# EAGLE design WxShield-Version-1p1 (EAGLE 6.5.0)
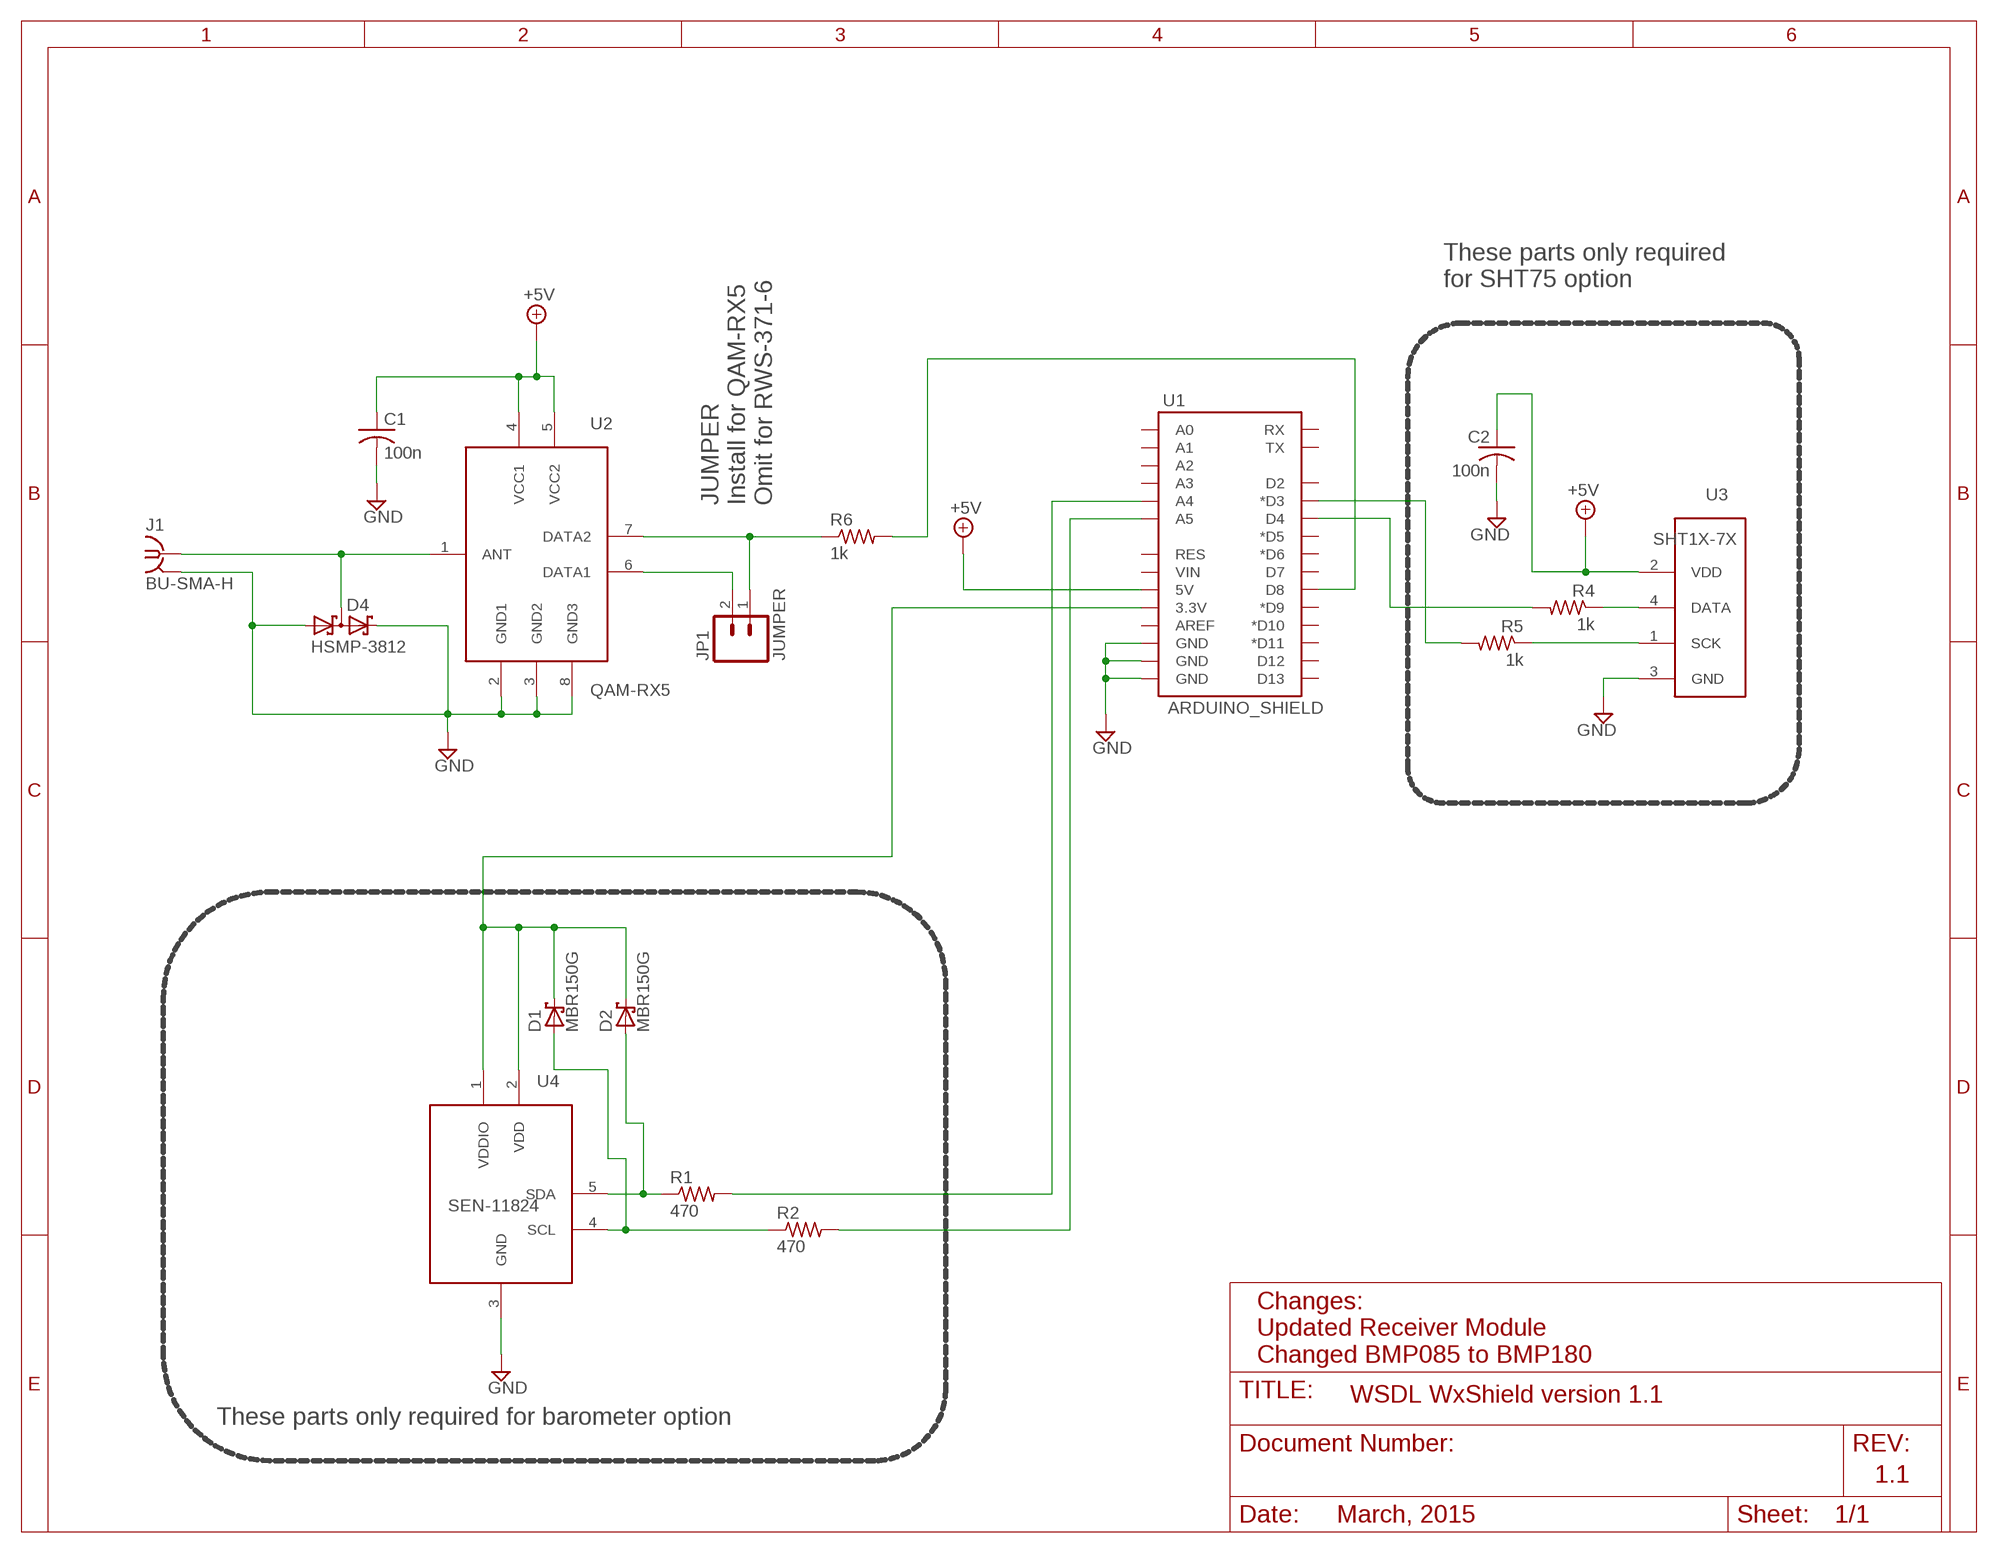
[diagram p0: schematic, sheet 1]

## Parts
C1  100n  C-US050-025X075  [C050-025X075]
C2  100n  C-US050-025X075  [C050-025X075]
D1  MBR150G  1N5817-B  [DO41-7.6]
D2  MBR150G  1N5817-B  [DO41-7.6]
D4  HSMP-3812  BAT30SW  [SOT323]
J1  BU-SMA-H  [BU-SMA-H]
JP1  JUMPER  M021X02_NO_SILK  [1X02_NO_SILK]
R1  470  R-US_0207/10  [0207/10]
R2  470  R-US_0207/10  [0207/10]
R4  1k  R-US_0207/10  [0207/10]
R5  1k  R-US_0207/10  [0207/10]
R6  1k  R-US_0207/10  [0207/10]
U1  ARDUINO_SHIELD  ARDUINO_SHIELDLABEL  [DUEMILANOVE_SHIELD]
U2  QAM-RX5  QAM-RX4  [QAM-RX4]
U3  SHT1X-7X  [SHT7X]
U4  SEN-11824  [SEN-11824]

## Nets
+5V: C1.1 C2.1 U1.5V U2.4(VCC1) U2.5(VCC2) U3.2(VDD)
GND: C1.2 C2.2 D4.1(A1) D4.2(C2) J1.2(GND) U1.GND@0(GND) U1.GND@1(GND) U1.GND@2(GND) U2.2(GND1) U2.3(GND2) U2.8(GND3) U3.3(GND) U4.3(GND)
N$1: JP1.1 R6.1 U2.7(DATA2)
N$2: JP1.2 U2.6(DATA1)
N$3: D2.A R1.1 U4.5(SDA)
N$4: D1.A R2.1 U4.4(SCL)
N$5: R1.2 U1.A4
N$6: R2.2 U1.A5
N$8: R4.1 U3.4(DATA)
N$9: R5.1 U3.1(SCK)
N$10: R5.2 U1.D3(*D3)
N$11: R4.2 U1.D4
N$12: R6.2 U1.D8
N$13: D1.C D2.C U1.3.3V U4.1(VDDIO) U4.2(VDD)
N$19: D4.3(C1A2) J1.1 U2.1(ANT)
Unconnected: U1.A0 U1.A1 U1.A2 U1.A3 U1.AREF U1.D2 U1.D5(*D5) U1.D6(*D6) U1.D7 U1.D9(*D9) U1.D10(*D10) U1.D11(*D11) U1.D12 U1.D13 U1.RES U1.RX U1.TX U1.VIN

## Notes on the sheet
- These parts only required
  for SHT75 option
- JUMPER
  Install for QAM-RX5
  Omit for RWS-371-6
- Changes:
  Updated Receiver Module
  Changed BMP085 to BMP180
- WSDL WxShield version 1.1
- These parts only required for barometer option
- 1.1
- March, 2015

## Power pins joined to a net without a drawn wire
GND: J1.3(GND) J1.4(GND) J1.5(GND)

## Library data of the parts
C1 C2 = resistor:C-US: CAPACITOR, American symbol
D1 D2 = diode:1N581*: 1.0A SCHOTTKY BARRIER RECTIFIER
D4 = max-local:BAT30SW: Dual Schottky diode Available in SOT-323 package
J1 = con-coax:BU-SMA-H: FEMALE SMA CONNECTOR Radiall
JP1 = SparkFun-Connectors:M02: Header 2
R1 R2 R4-R6 = resistor:R-US_: RESISTOR, American symbol
U1 = SparkFun-Boards:ARDUINO_SHIELD: Arduino shield footprint
U2 = max-local:QAM-RX4: RF Solutions OOK Receiver Module
U3 = max-local:SHT1X
U4 = max-local:SEN-11824: SparkFun BMP180 Breakout Board

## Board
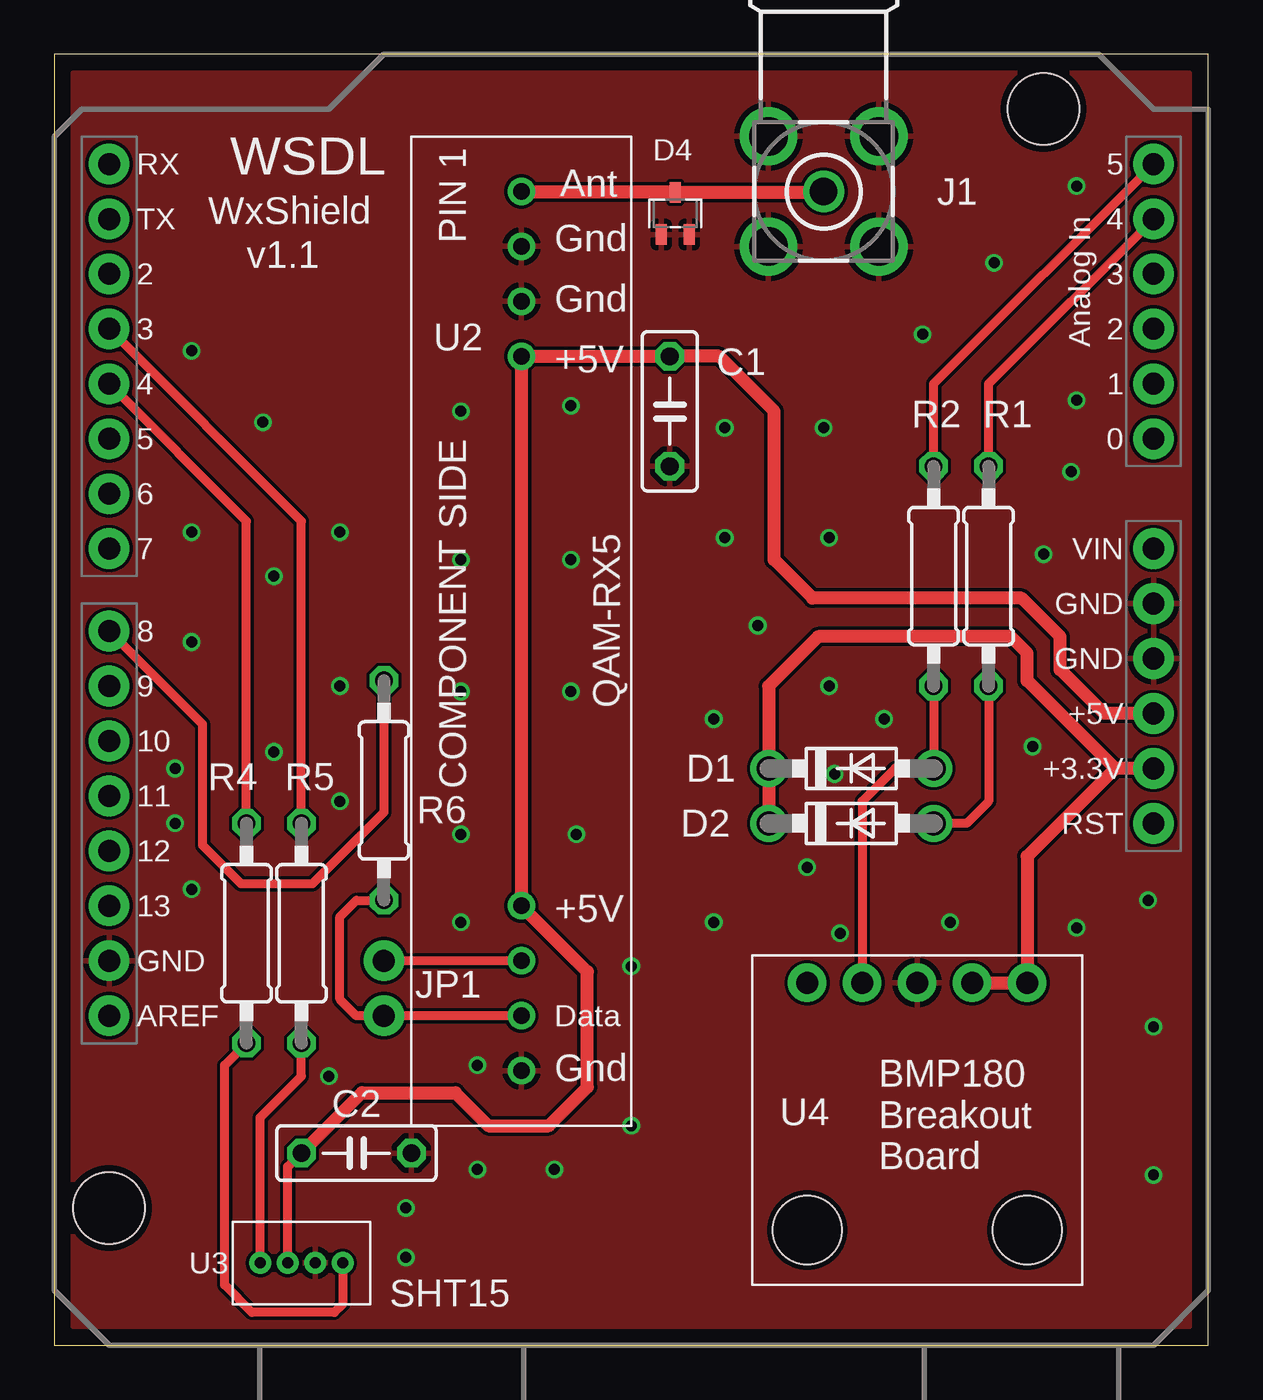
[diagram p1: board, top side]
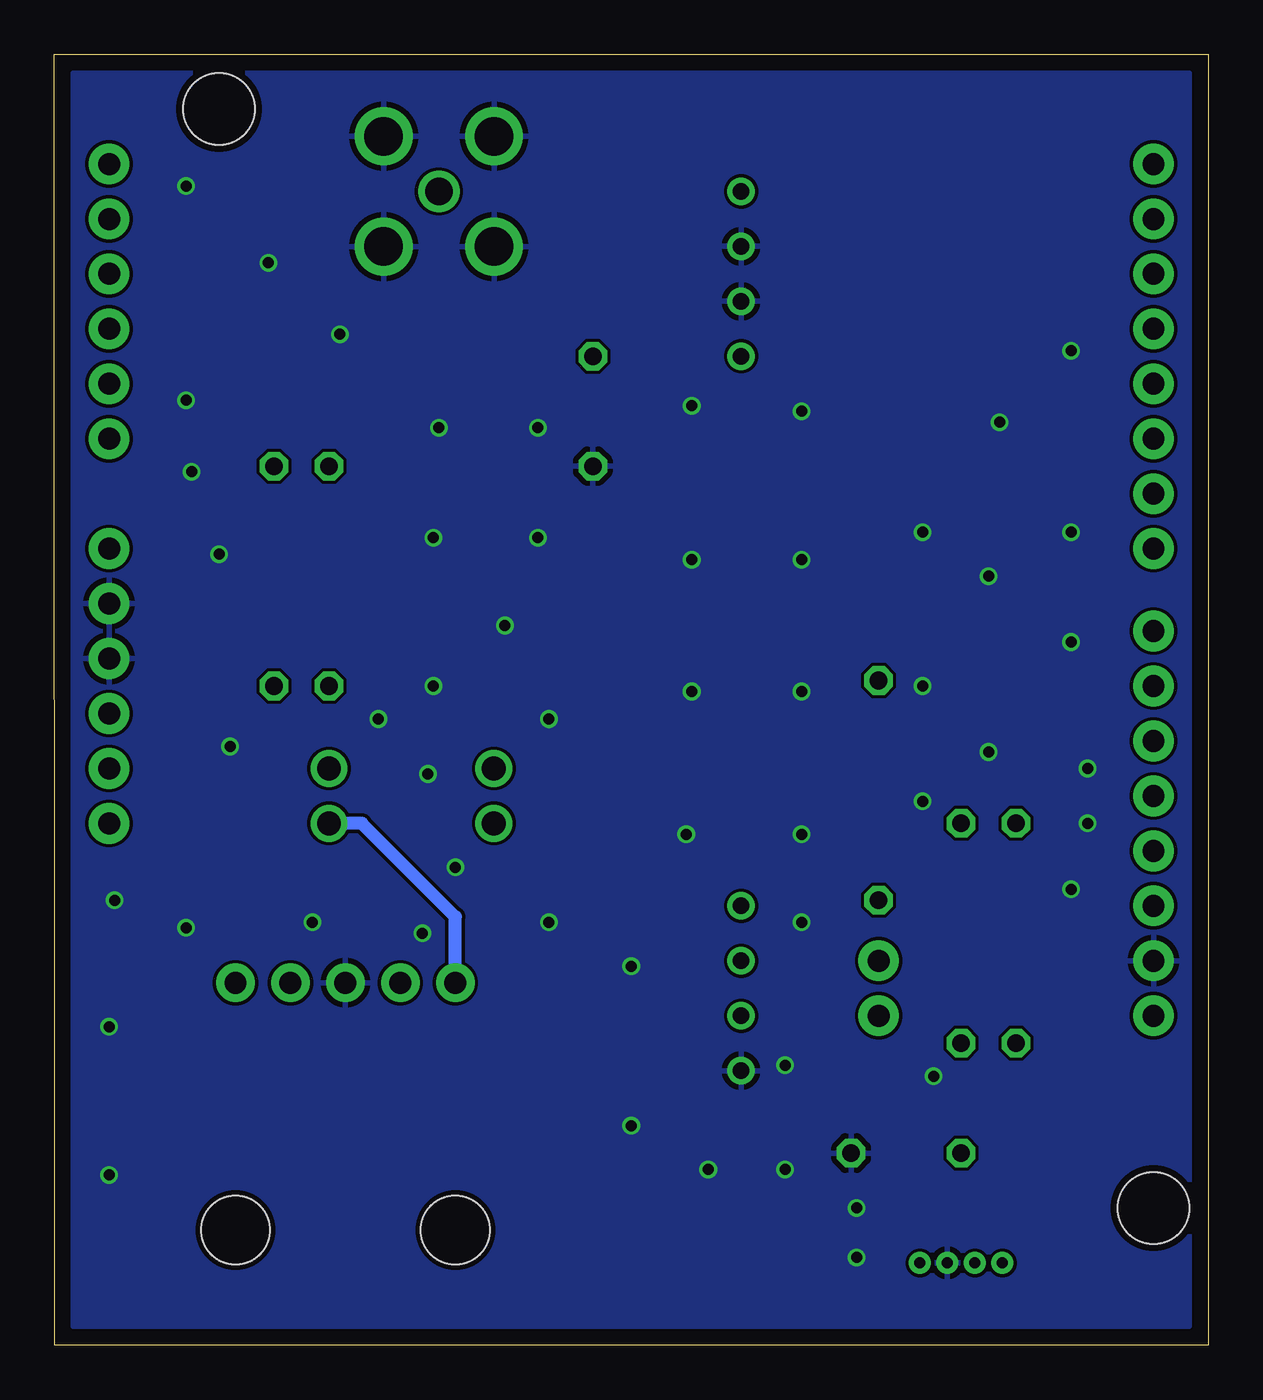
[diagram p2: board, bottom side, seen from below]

Size 53.34 x 59.69 mm. Coordinates in mm from the lower left corner, seen from the top.
Outline: 0,0 53.32,0 53.34,59.69 0,59.69 0,0
Copper layers (1*16): Top 0.035mm / dielectric 1.5mm / Bottom 0.035mm
Design rules "SeeedStudio_2layer_DRU_no_angle_20140221": minimum track width 6mil, minimum drill 12mil, track to track 6mil, track to pad 6mil, pad to pad 6mil, via to via 6mil, smd to smd 0mil, copper to edge 10mil, drill to drill 10mil, minimum pad ring 10mil, minimum via ring 6mil, stop-mask expansion 2mil, vias tented up to drill 100mil, thermal gap 10mil

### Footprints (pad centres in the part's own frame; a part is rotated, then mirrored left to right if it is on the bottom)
C050-025X075 = drill 0.813 octagon: 1 -2.54,0; 2 2.54,0
DO41-7.6 = drill 1.1 pad 1.7: A 3.81,0; C -3.81,0
SOT323 = smd 0.5 x 0.95: 1 -0.65,-0.975; 2 0.65,-0.975; 3 0,0.975
BU-SMA-H = drill 1.27: 1 0,0 | drill 1.778: 2 -2.55,2.55; 3 2.55,2.55; 4 2.55,-2.55; 5 -2.55,-2.55
1X02_NO_SILK = drill 1.016 pad 1.88: 1 0,0; 2 2.54,0
0207/10 = drill 0.813 octagon: 1 -5.08,0; 2 5.08,0
DUEMILANOVE_SHIELD = drill 1.016 pad 1.88: 3.3V 50.8,26.67; 5V 50.8,29.21; A0 50.8,41.91; A1 50.8,44.45; A2 50.8,46.99; A3 50.8,49.53; A4 50.8,52.07; A5 50.8,54.61; AREF 2.54,15.24; D2 2.54,49.53; D3 2.54,46.99; D4 2.54,44.45; D5 2.54,41.91; D6 2.54,39.37; D7 2.54,36.83; D8 2.54,33.02; D9 2.54,30.48; D10 2.54,27.94; D11 2.54,25.4; D12 2.54,22.86; D13 2.54,20.32; GND@0 50.8,31.75; GND@1 50.8,34.29; GND@2 2.54,17.78; RES 50.8,24.13; RX 2.54,54.61; TX 2.54,52.07; VIN 50.8,36.83 | hole 3.302: 45.72,57.15; 2.54,6.35
QAM-RX4 = drill 0.762: 1 -20.32,0; 2 -17.78,0; 3 -15.24,0; 4 -12.7,0; 5 12.7,0; 6 15.24,0; 7 17.78,0; 8 20.32,0
SHT7X = drill 0.508 pad 1.016: 1 -1.905,0; 2 -0.635,0; 3 0.635,0; 4 1.905,0
SEN-11824 = drill 1.016 pad 1.778: 1 5.08,6.35; 2 2.54,6.35; 3 0,6.35; 4 -2.54,6.35; 5 -5.08,6.35 | hole 3.175: -5.08,-5.08; 5.08,-5.08

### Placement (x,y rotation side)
C1  28.45,43.18 270 top
C2  13.97,8.89 0 top
D1  36.83,26.67 0 top
D2  36.83,24.13 0 top
D4  28.7,52.32 0 top
J1  35.56,53.34 90 top
JP1  15.24,15.24 90 top
R1  43.18,35.56 90 top
R2  40.64,35.56 90 top
R4  8.89,19.05 90 top
R5  11.43,19.05 90 top
R6  15.24,25.65 90 top
U1  0,0 0 top
U2  21.59,33.02 270 top
U3  11.43,3.81 0 top
U4  39.88,10.41 0 top

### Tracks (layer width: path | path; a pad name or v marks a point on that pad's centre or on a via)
+5V
  Top 0.406: U3.2 10.79,8.26 C2.1
  Top 0.61: U1.5V 48.51,29.21 46.48,31.24 46.48,32.77 44.7,34.54 35.05,34.54 33.27,36.32 33.27,43.18 30.73,45.72 C1.1 U2.4 U2.5 24.64,17.27 24.64,11.94 22.86,10.16 20.07,10.16 18.54,11.68 14.22,11.68 C2.1
GND  (via drill 0.51)
  other vias: 12.7,12.45 19.56,12.95 19.56,8.13 23.11,8.13 26.67,10.16 26.67,17.53 24.13,23.62 18.8,23.62 18.8,19.56 23.88,30.23 18.8,30.23 18.8,36.32 23.88,36.32 23.88,43.43 18.8,43.18 6.35,32.51 6.35,37.59 10.16,27.43 10.16,35.56 30.99,42.42 30.99,37.34 35.81,37.34 35.56,42.42 35.81,30.48 36.07,26.42 34.8,22.1 36.32,19.05 30.48,19.56 30.48,28.96 32.51,33.27 47.24,43.69 40.13,46.74 47.24,53.59 43.43,50.04 46.99,40.39 45.72,36.58 50.55,20.57 50.8,14.73 50.8,7.87 16.26,4.06 16.26,6.35 45.21,27.69 38.35,28.96 47.24,19.3 41.4,19.56 13.21,25.15 13.21,30.48 13.21,37.59 6.35,45.97 9.65,42.67 5.59,26.67 5.59,24.13 6.35,21.08
  pour Top: 0.89,0.89 52.45,0.89 52.45,58.8 0.89,58.8
  pour Bottom: 0.89,0.89 52.45,0.89 52.45,58.8 0.89,58.8
N$1
  Top 0.406: U2.7 JP1.1 13.97,15.24 13.21,16 13.21,19.81 13.97,20.57 R6.1
N$2
  Top 0.406: U2.6 JP1.2
N$3
  Top 0.406: R1.1 43.18,25.15 42.16,24.13 D2.A
  Bottom 0.61: U4.5 34.8,19.81 39.12,24.13 D2.A
N$4
  Top 0.406: R2.1 D1.A 38.86,26.67 37.34,25.15 U4.4
N$5
  Top 0.406: R1.2 43.18,44.45 U1.A4
N$6
  Top 0.406: R2.2 40.64,44.45 U1.A5
N$8
  Top 0.406: U3.4 13.34,1.91 12.95,1.52 9.14,1.52 7.87,2.79 7.87,12.95 R4.1
N$9
  Top 0.406: U3.1 9.53,10.54 11.43,12.45 R5.1
N$10
  Top 0.406: R5.2 11.43,38.1 U1.D3
N$11
  Top 0.406: R4.2 8.89,38.1 U1.D4
N$12
  Top 0.406: R6.2 15.24,24.64 11.94,21.34 8.64,21.34 6.86,23.11 6.86,28.7 U1.D8
N$13
  Top 0.61: U1.3.3V 49.02,26.67 | 49.02,26.67 44.96,30.73 44.96,32 44.2,32.77 35.31,32.77 33.02,30.48 D1.C D2.C | U4.2 U4.1 44.96,22.61 49.02,26.67
N$19
  Top 0.61: U2.1 21.63,53.3 D4.3 35.52,53.3 J1.1

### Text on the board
tPlace: WSDL | Ant | WxShield | Gnd | v1.1 | Gnd | +5V | +5V | Data | Gnd | BMP180 / Breakout / Board | SHT15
